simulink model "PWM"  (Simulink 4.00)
settings: Solver=ode5  StartTime=0.0  StopTime=0.002  FixedStep=0.00001  RelTol=1e-3
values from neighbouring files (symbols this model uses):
  Fpwm = 5000    [GNM_lsg_ini.m]
  Umax = 200    [GNM_lsg_ini.m]
libraries: simulink3 x1

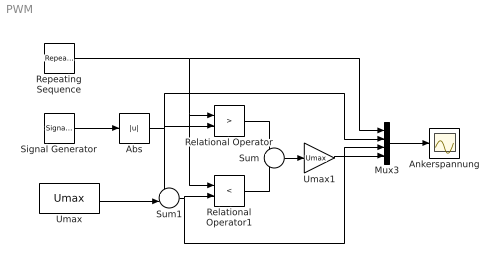
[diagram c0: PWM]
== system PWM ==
  Abs : Abs  SaturateOnIntegerOverflow=on
  Ankerspannung : Scope
  Mux3 : Mux  Inputs=4
  Relational Operator : RelationalOperator  Operator=>
  Relational Operator1 : RelationalOperator  Operator=<
  Repeating Sequence : simulink3/Sources/Repeating Sequence  rep_seq_t=[0 2.1] * 0.001  rep_seq_y=[0.9 -0.4] * Umax
  Signal Generator : SignalGenerator  WaveForm=sawtooth  Amplitude=Umax  Frequency=Fpwm  Units=Hertz
  Sum : Sum  Inputs=+-  SaturateOnIntegerOverflow=on
  Sum1 : Sum  Inputs=+-|  SaturateOnIntegerOverflow=on
  Umax : Constant  Value=Umax
  Umax1 : Gain  Gain=Umax  Multiplication=Element-wise(K.*u)  SaturateOnIntegerOverflow=on
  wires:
  Repeating Sequence/1 -> Relational Operator/1, Relational Operator1/1, Mux3/1
  Abs/1 -> Sum1/1, Relational Operator/2, Mux3/2
  Umax/1 -> Sum1/2
  Relational Operator/1 -> Sum/1
  Relational Operator1/1 -> Sum/2
  Sum/1 -> Umax1/1
  Mux3/1 -> Ankerspannung/1
  Umax1/1 -> Mux3/4
  Sum1/1 -> Relational Operator1/2, Mux3/3
  Signal Generator/1 -> Abs/1
